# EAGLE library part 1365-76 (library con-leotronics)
DUAL ROW STRAIGHT HEADER 1364 SERIES. 1.27mm x 1.27mm. Without Fixing Post. SMT Source: http://www.leotronics.co.uk/Conexcon/Data%20Sheets/sec.%20A/1364ing.pdf
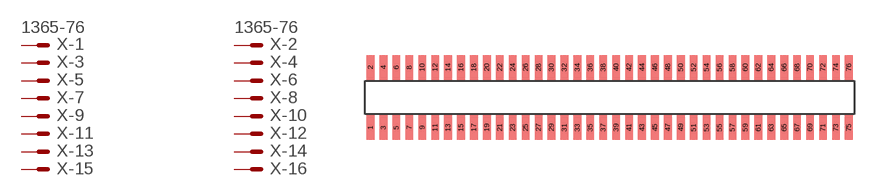
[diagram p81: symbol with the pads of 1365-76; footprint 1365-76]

Designator prefix X; gates -1=MVAL -2=MVAL -3=M -4=M -5=M -6=M -7=M -8=M -9=M -10=M -11=M -12=M -13=M -14=M -15=M -16=M -17=M -18=M -19=M -20=M -21=M -22=M -23=M -24=M -25=M -26=M -27=M -28=M -29=M -30=M -31=M -32=M -33=M -34=M -35=M -36=M -37=M -38=M -39=M -40=M -41=M -42=M -43=M -44=M -45=M -46=M -47=M -48=M -49=M -50=M -51=M -52=M -53=M -54=M -55=M -56=M -57=M -58=M -59=M -60=M -61=M -62=M -63=M -64=M -65=M -66=M -67=M -68=M -69=M -70=M -71=M -72=M -73=M -74=M -75=M -76=M

## 1365-76 (OC_FARNELL: unknown; OC_NEWARK: unknown)  [1365-76]
1  -1:S  pas
2  -2:S  pas
3  -3:S  pas
4  -4:S  pas
5  -5:S  pas
6  -6:S  pas
7  -7:S  pas
8  -8:S  pas
9  -9:S  pas
10  -10:S  pas
11  -11:S  pas
12  -12:S  pas
13  -13:S  pas
14  -14:S  pas
15  -15:S  pas
16  -16:S  pas
17  -17:S  pas
18  -18:S  pas
19  -19:S  pas
20  -20:S  pas
21  -21:S  pas
22  -22:S  pas
23  -23:S  pas
24  -24:S  pas
25  -25:S  pas
26  -26:S  pas
27  -27:S  pas
28  -28:S  pas
29  -29:S  pas
30  -30:S  pas
31  -31:S  pas
32  -32:S  pas
33  -33:S  pas
34  -34:S  pas
35  -35:S  pas
36  -36:S  pas
37  -37:S  pas
38  -38:S  pas
39  -39:S  pas
40  -40:S  pas
41  -41:S  pas
42  -42:S  pas
43  -43:S  pas
44  -44:S  pas
45  -45:S  pas
46  -46:S  pas
47  -47:S  pas
48  -48:S  pas
49  -49:S  pas
50  -50:S  pas
51  -51:S  pas
52  -52:S  pas
53  -53:S  pas
54  -54:S  pas
55  -55:S  pas
56  -56:S  pas
57  -57:S  pas
58  -58:S  pas
59  -59:S  pas
60  -60:S  pas
61  -61:S  pas
62  -62:S  pas
63  -63:S  pas
64  -64:S  pas
65  -65:S  pas
66  -66:S  pas
67  -67:S  pas
68  -68:S  pas
69  -69:S  pas
70  -70:S  pas
71  -71:S  pas
72  -72:S  pas
73  -73:S  pas
74  -74:S  pas
75  -75:S  pas
76  -76:S  pas

## Footprint 1365-76 (pad centres in mm)
DUAL ROW STRAIGHT HEADER 1364 SERIES. 1.27mm x 1.27mm. Without Fixing Post. SMT Source: http://www.leotronics.co.uk/Conexcon/Data%20Sheets/sec.%20A/1364ing.pdf
smd 0.76 x 2.4: 1 -23.495,-2.95; 2 -23.495,2.95; 3 -22.225,-2.95; 4 -22.225,2.95; 5 -20.955,-2.95; 6 -20.955,2.95; 7 -19.685,-2.95; 8 -19.685,2.95; 9 -18.415,-2.95; 10 -18.415,2.95; 11 -17.145,-2.95; 12 -17.145,2.95; 13 -15.875,-2.95; 14 -15.875,2.95; 15 -14.605,-2.95; 16 -14.605,2.95; 17 -13.335,-2.95; 18 -13.335,2.95; 19 -12.065,-2.95; 20 -12.065,2.95; 21 -10.795,-2.95; 22 -10.795,2.95; 23 -9.525,-2.95; 24 -9.525,2.95; 25 -8.255,-2.95; 26 -8.255,2.95; 27 -6.985,-2.95; 28 -6.985,2.95; 29 -5.715,-2.95; 30 -5.715,2.95; 31 -4.445,-2.95; 32 -4.445,2.95; 33 -3.175,-2.95; 34 -3.175,2.95; 35 -1.905,-2.95; 36 -1.905,2.95; 37 -0.635,-2.95; 38 -0.635,2.95; 39 0.635,-2.95; 40 0.635,2.95; 41 1.905,-2.95; 42 1.905,2.95; 43 3.175,-2.95; 44 3.175,2.95; 45 4.445,-2.95; 46 4.445,2.95; 47 5.715,-2.95; 48 5.715,2.95; 49 6.985,-2.95; 50 6.985,2.95; 51 8.255,-2.95; 52 8.255,2.95; 53 9.525,-2.95; 54 9.525,2.95; 55 10.795,-2.95; 56 10.795,2.95; 57 12.065,-2.95; 58 12.065,2.95; 59 13.335,-2.95; 60 13.335,2.95; 61 14.605,-2.95; 62 14.605,2.95; 63 15.875,-2.95; 64 15.875,2.95; 65 17.145,-2.95; 66 17.145,2.95; 67 18.415,-2.95; 68 18.415,2.95; 69 19.685,-2.95; 70 19.685,2.95; 71 20.955,-2.95; 72 20.955,2.95; 73 22.225,-2.95; 74 22.225,2.95; 75 23.495,-2.95; 76 23.495,2.95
